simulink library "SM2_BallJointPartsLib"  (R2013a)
settings: Solver=ode45  StartTime=0.0  StopTime=10.0  RelTol=1e-3
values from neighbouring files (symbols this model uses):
  m = v*BEAM.rho    [FlexBeamModelConstruct2.m]    (also in FlexBeamModelConstruct3.m = BEAM.rho*v; FlexBeam_1D_Construct.m = REF.m/REF.l*a.*(linspace(1-OPT.MassBiais+1e-6,1+OPT.MassBiai; FlexBeam_3D_Construct.m = REF.m/REF.l*a.*(linspace(1-OPT.MassBiais+1e-6,1+OPT.MassBiai; FreeFlexBeam_3D_Construct.m = REF.m/REF.l*a.*tmp2)
  N = D(1)+(H4^2+H3^2)/H2^2-(E(1)*H4+F(1)*H3)/H2    [MGD.m]    (also in MGD2.m)
  s = -sign(imag(KGZ_fr_tmp))    [LinprogReguliOptimFunc_1.m]    (also in LinprogReguliOptimFunc_2.m; LinprogReguliOptimFunc_1 - Copie.m)
  X = cos(phi(i))*x+sin(phi(i))*y    [MGI.m]
  Y = fft(y(:,i),NFFT)/L    [fft_bis.m]    (also in MGI.m = -sin(phi(i))*x+cos(phi(i))*y)
  Z = z    [MGI.m]
undefined symbols (not defined in the file or in its folder): AxisID, deg, rad, SimParam
libraries: sm_lib x15

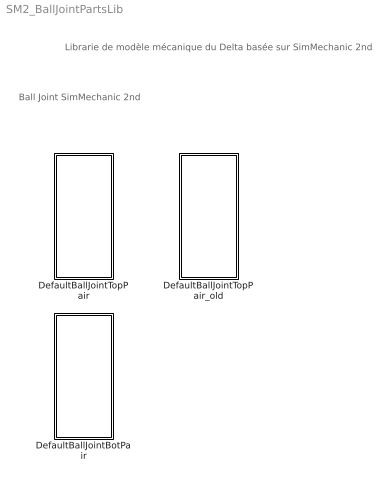
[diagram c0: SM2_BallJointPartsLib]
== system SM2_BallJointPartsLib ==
  note: Librarie de modèle mécanique du Delta basée sur SimMechanic 2nd
  note: Ball Joint SimMechanic 2nd
  DefaultBallJointBotPair : Subsystem  InitFcn=SimParam.BallJoint = Balljoint_paramInitFnc(RawParam);
  DefaultBallJointTopPair : Subsystem  InitFcn=SimParam.BallJoint = Balljoint_paramInitFnc(RawParam);
  DefaultBallJointTopPair_old : Subsystem  InitFcn=SimParam.BallJoint = Balljoint_paramInitFnc(RawParam);

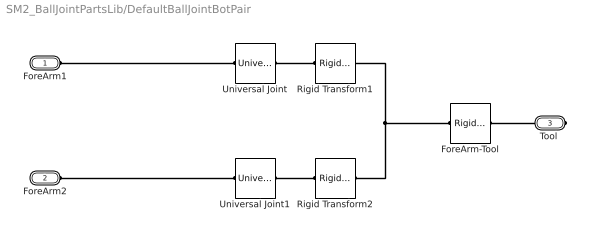
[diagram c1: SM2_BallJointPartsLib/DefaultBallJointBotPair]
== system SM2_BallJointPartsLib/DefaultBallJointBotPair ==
  ForeArm-Tool : sm_lib/Frames and  Transforms/Rigid  Transform  TranslationMethod=Cylindrical  TranslationLengthUnit=m  TranslationStandardAxis=+Z  TranslationStandardOffset=0  TranslationCartesianOffset=[-SimParam.BallJoint.r 0 0]  TranslationROffset=SimParam.BallJoint.r  TranslationROffsetUnits=m  TranslationZOffset=0  TranslationZOffsetUnits=m  TranslationThetaOffset=SimParam.BallJoint.Theta(AxisID)  TranslationThetaOffsetUnits=rad  RotationMethod=StandardAxis  RotationAngleUnits=rad  RotationStandardAxis=+Z  RotationAngle=SimParam.BallJoint.Theta(AxisID)  RotationArbitraryAxis=[1,1,1]  FollAlignAxisA=+X  BaseAlignAxisA=+Y  FollAlignAxisB=+Y  BaseAlignAxisB=+Z  BlockFunction=simmechanics.library.frames_transforms.rigid_transform
  Rigid Transform1 : sm_lib/Frames and  Transforms/Rigid  Transform  TranslationMethod=Cartesian  TranslationLengthUnit=m  TranslationStandardAxis=+Z  TranslationStandardOffset=0  TranslationCartesianOffset=[0 SimParam.BallJoint.d(2) 0]  TranslationROffset=0.2  TranslationROffsetUnits=m  TranslationZOffset=0  TranslationZOffsetUnits=m  TranslationThetaOffset=0  TranslationThetaOffsetUnits=deg  RotationMethod=None  RotationAngleUnits=rad  RotationStandardAxis=+Y  RotationAngle=0.2  RotationArbitraryAxis=[0 0 1]  FollAlignAxisA=+Z  BaseAlignAxisA=+Y  FollAlignAxisB=+X  BaseAlignAxisB=+X  BlockFunction=simmechanics.library.frames_transforms.rigid_transform
  Rigid Transform2 : sm_lib/Frames and  Transforms/Rigid  Transform  TranslationMethod=Cartesian  TranslationLengthUnit=m  TranslationStandardAxis=+Z  TranslationStandardOffset=0  TranslationCartesianOffset=[0 -SimParam.BallJoint.d(1) 0]  TranslationROffset=0.2  TranslationROffsetUnits=m  TranslationZOffset=0  TranslationZOffsetUnits=m  TranslationThetaOffset=0  TranslationThetaOffsetUnits=deg  RotationMethod=None  RotationAngleUnits=rad  RotationStandardAxis=+Y  RotationAngle=0.2  RotationArbitraryAxis=[0 0 1]  FollAlignAxisA=+Z  BaseAlignAxisA=+Y  FollAlignAxisB=+X  BaseAlignAxisB=+X  BlockFunction=simmechanics.library.frames_transforms.rigid_transform
  Universal Joint : sm_lib/Joints/Universal  Joint  SenseConstraintForceX=off  SenseConstraintForceY=off  SenseConstraintForceZ=off  SenseConstraintTorqueX=off  SenseConstraintTorqueY=off  SenseConstraintTorqueZ=off  ConstraintWrenchDir=FollowerOnBase  ConstraintWrenchFrame=BaseFrame  RxEquilibriumPosition=0  RxEquilibriumPositionUnits=deg  RxSpringStiffness=0  RxSpringStiffnessUnits=N*m/deg  RxDampingCoefficient=SimParam.BallJoint.c  RxDampingCoefficientUnits=N*m/(rad/s)  RxActuationMode=NoActuation  RxSensePosition=off  RxSenseVelocity=off  RxSenseAcceleration=off  RxSenseTorqueForce=off  RxPositionTargetValue=0  RxPositionTargetValueUnits=deg  RxPositionTargetSpecify=off  RxPositionTargetPriority=High  RxVelocityTargetValue=0  RxVelocityTargetValueUnits=deg/s  RxVelocityTargetSpecify=off  RxVelocityTargetPriority=High  RyEquilibriumPosition=0  RyEquilibriumPositionUnits=deg  RySpringStiffness=0  RySpringStiffnessUnits=N*m/deg  RyDampingCoefficient=SimParam.BallJoint.c  RyDampingCoefficientUnits=N*m/(rad/s)  RyActuationMode=NoActuation  RySensePosition=off  RySenseVelocity=off  RySenseAcceleration=off  RySenseTorqueForce=off  RyPositionTargetValue=0  RyPositionTargetValueUnits=deg  RyPositionTargetSpecify=off  RyPositionTargetPriority=High  RyVelocityTargetValue=0  RyVelocityTargetValueUnits=deg/s  RyVelocityTargetSpecify=off  RyVelocityTargetPriority=High  BlockFunction=simmechanics.library.joints.universal_joint
  Universal Joint1 : sm_lib/Joints/Universal  Joint  SenseConstraintForceX=off  SenseConstraintForceY=off  SenseConstraintForceZ=off  SenseConstraintTorqueX=off  SenseConstraintTorqueY=off  SenseConstraintTorqueZ=off  ConstraintWrenchDir=FollowerOnBase  ConstraintWrenchFrame=BaseFrame  RxEquilibriumPosition=0  RxEquilibriumPositionUnits=deg  RxSpringStiffness=0  RxSpringStiffnessUnits=N*m/deg  RxDampingCoefficient=SimParam.BallJoint.c  RxDampingCoefficientUnits=N*m/(rad/s)  RxActuationMode=NoActuation  RxSensePosition=off  RxSenseVelocity=off  RxSenseAcceleration=off  RxSenseTorqueForce=off  RxPositionTargetValue=0  RxPositionTargetValueUnits=deg  RxPositionTargetSpecify=off  RxPositionTargetPriority=High  RxVelocityTargetValue=0  RxVelocityTargetValueUnits=deg/s  RxVelocityTargetSpecify=off  RxVelocityTargetPriority=High  RyEquilibriumPosition=0  RyEquilibriumPositionUnits=deg  RySpringStiffness=0  RySpringStiffnessUnits=N*m/deg  RyDampingCoefficient=SimParam.BallJoint.c  RyDampingCoefficientUnits=N*m/(rad/s)  RyActuationMode=NoActuation  RySensePosition=off  RySenseVelocity=off  RySenseAcceleration=off  RySenseTorqueForce=off  RyPositionTargetValue=0  RyPositionTargetValueUnits=deg  RyPositionTargetSpecify=off  RyPositionTargetPriority=High  RyVelocityTargetValue=0  RyVelocityTargetValueUnits=deg/s  RyVelocityTargetSpecify=off  RyVelocityTargetPriority=High  BlockFunction=simmechanics.library.joints.universal_joint
  ForeArm1 : PMIOPort  Port=1  Side=Left
  ForeArm2 : PMIOPort  Port=2  Side=Left
  "Tool " : PMIOPort  Port=3  Side=Right
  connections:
  Universal Joint/LConn1 -- ForeArm1/RConn1
  Universal Joint1/LConn1 -- ForeArm2/RConn1
  ForeArm-Tool/LConn1 -- "Tool "/RConn1
  Rigid Transform2/LConn1 -- Rigid Transform1/LConn1 -- ForeArm-Tool/RConn1
  Rigid Transform2/RConn1 -- Universal Joint1/RConn1
  Rigid Transform1/RConn1 -- Universal Joint/RConn1

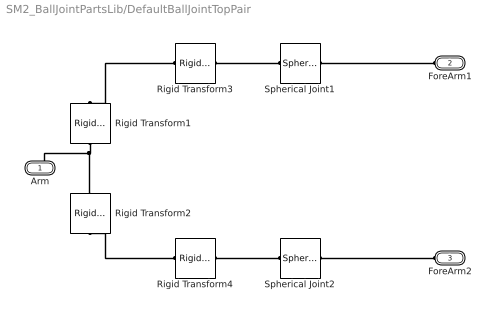
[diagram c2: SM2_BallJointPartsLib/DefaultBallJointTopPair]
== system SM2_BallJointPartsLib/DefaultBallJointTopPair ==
  Rigid Transform1 : sm_lib/Frames and  Transforms/Rigid  Transform  TranslationMethod=Cartesian  TranslationLengthUnit=m  TranslationStandardAxis=+Z  TranslationStandardOffset=0  TranslationCartesianOffset=[0 SimParam.BallJoint.d(1) 0]  TranslationROffset=0.2  TranslationROffsetUnits=m  TranslationZOffset=0  TranslationZOffsetUnits=m  TranslationThetaOffset=0  TranslationThetaOffsetUnits=deg  RotationMethod=None  RotationAngleUnits=rad  RotationStandardAxis=+Y  RotationAngle=0.2  RotationArbitraryAxis=[0 0 1]  FollAlignAxisA=+Z  BaseAlignAxisA=+Y  FollAlignAxisB=+X  BaseAlignAxisB=+X  BlockFunction=simmechanics.library.frames_transforms.rigid_transform
  Rigid Transform2 : sm_lib/Frames and  Transforms/Rigid  Transform  TranslationMethod=Cartesian  TranslationLengthUnit=m  TranslationStandardAxis=+Z  TranslationStandardOffset=0  TranslationCartesianOffset=[0 -SimParam.BallJoint.d(2) 0]  TranslationROffset=0.2  TranslationROffsetUnits=m  TranslationZOffset=0  TranslationZOffsetUnits=m  TranslationThetaOffset=0  TranslationThetaOffsetUnits=deg  RotationMethod=None  RotationAngleUnits=rad  RotationStandardAxis=+Y  RotationAngle=0.2  RotationArbitraryAxis=[0 0 1]  FollAlignAxisA=+Z  BaseAlignAxisA=+Y  FollAlignAxisB=+X  BaseAlignAxisB=+X  BlockFunction=simmechanics.library.frames_transforms.rigid_transform
  Rigid Transform3 : sm_lib/Frames and  Transforms/Rigid  Transform  TranslationMethod=None  TranslationLengthUnit=m  TranslationStandardAxis=+Z  TranslationStandardOffset=0  TranslationCartesianOffset=[0 -SimParam.BallJoint.d(2) 0]  TranslationROffset=0.2  TranslationROffsetUnits=m  TranslationZOffset=0  TranslationZOffsetUnits=m  TranslationThetaOffset=0  TranslationThetaOffsetUnits=deg  RotationMethod=ArbitraryAxis  RotationAngleUnits=rad  RotationStandardAxis=+Y  RotationAngle=SimParam.IC.ArmForeArmRotAng(AxisID)  RotationArbitraryAxis=SimParam.IC.ArmForeArmRotVec(AxisID,:)  FollAlignAxisA=+Z  BaseAlignAxisA=+Y  FollAlignAxisB=+X  BaseAlignAxisB=+X  BlockFunction=simmechanics.library.frames_transforms.rigid_transform
  Rigid Transform4 : sm_lib/Frames and  Transforms/Rigid  Transform  TranslationMethod=None  TranslationLengthUnit=m  TranslationStandardAxis=+Z  TranslationStandardOffset=0  TranslationCartesianOffset=[0 -SimParam.BallJoint.d(2) 0]  TranslationROffset=0.2  TranslationROffsetUnits=m  TranslationZOffset=0  TranslationZOffsetUnits=m  TranslationThetaOffset=0  TranslationThetaOffsetUnits=deg  RotationMethod=ArbitraryAxis  RotationAngleUnits=rad  RotationStandardAxis=+Y  RotationAngle=SimParam.IC.ArmForeArmRotAng(AxisID)  RotationArbitraryAxis=SimParam.IC.ArmForeArmRotVec(AxisID,:)  FollAlignAxisA=+Z  BaseAlignAxisA=+Y  FollAlignAxisB=+X  BaseAlignAxisB=+X  BlockFunction=simmechanics.library.frames_transforms.rigid_transform
  Spherical Joint1 : sm_lib/Joints/Spherical  Joint  SenseConstraintForceX=off  SenseConstraintForceY=off  SenseConstraintForceZ=off  SenseConstraintTorqueX=off  SenseConstraintTorqueY=off  SenseConstraintTorqueZ=off  ConstraintWrenchDir=FollowerOnBase  ConstraintWrenchFrame=BaseFrame  DefPosRotationMethod=None  DefPosRotationAngleUnits=deg  DefPosRotationStandardAxis=+Z  DefPosRotationAngle=0  DefPosRotationArbitraryAxis=[0 0 1]  DefPosFollAlignAxisA=+X  DefPosBaseAlignAxisA=+Y  DefPosFollAlignAxisB=+Y  DefPosBaseAlignAxisB=+Z  EqPosRotationMethod=None  EqPosRotationAngleUnits=deg  EqPosRotationStandardAxis=+Z  EqPosRotationAngle=0  EqPosRotationArbitraryAxis=[0 0 1]  EqPosFollAlignAxisA=+X  EqPosBaseAlignAxisA=+Y  EqPosFollAlignAxisB=+Y  EqPosBaseAlignAxisB=+Z  SpringStiffness=0  SpringStiffnessUnits=N*m/deg  DampingCoefficient=SimParam.BallJoint.c  DampingCoefficientUnits=N*m/(rad/s)  ActuateTorqueX=off  ActuateTorqueY=off  ActuateTorqueZ=off  ActuateTorque=off  ActuationMode=NoActuation  ActuationFrame=BaseFrame  SensePosition=off  SenseVelocityX=off  SenseVelocityY=off  SenseVelocityZ=off  SenseVelocity=off  SenseAccelerationX=off  SenseAccelerationY=off  SenseAccelerationZ=off  SenseAcceleration=off  SenseTorqueX=off  SenseTorqueY=off  SenseTorqueZ=off  SenseTorqueForce=off  SensingFrame=BaseFrame  PositionTargetRotationMethod=StandardAxis  PositionTargetRotationAngleUnits=rad  PositionTargetRotationStandardAxis=+Z  PositionTargetRotationAngle=0  PositionTargetRotationArbitraryAxis=SimParam.IC.ArmForeArmRotVec(AxisID,:)  PositionTargetFollAlignAxisA=+X  PositionTargetBaseAlignAxisA=+Y  PositionTargetFollAlignAxisB=+Y  PositionTargetBaseAlignAxisB=+Z  PositionTargetSpecify=off  PositionTargetPriority=Low  VelocityTargetValue=[0 0 0]  VelocityTargetValueUnits=rad/s  VelocityTargetSpecify=on  VelocityTargetPriority=High  VelocityTargetInFollowerFrame=on  BlockFunction=simmechanics.library.joints.spherical_joint
  Spherical Joint2 : sm_lib/Joints/Spherical  Joint  SenseConstraintForceX=off  SenseConstraintForceY=off  SenseConstraintForceZ=off  SenseConstraintTorqueX=off  SenseConstraintTorqueY=off  SenseConstraintTorqueZ=off  ConstraintWrenchDir=FollowerOnBase  ConstraintWrenchFrame=BaseFrame  DefPosRotationMethod=None  DefPosRotationAngleUnits=deg  DefPosRotationStandardAxis=+Z  DefPosRotationAngle=0  DefPosRotationArbitraryAxis=[0 0 1]  DefPosFollAlignAxisA=+X  DefPosBaseAlignAxisA=+Y  DefPosFollAlignAxisB=+Y  DefPosBaseAlignAxisB=+Z  EqPosRotationMethod=None  EqPosRotationAngleUnits=deg  EqPosRotationStandardAxis=+Z  EqPosRotationAngle=0  EqPosRotationArbitraryAxis=[0 0 1]  EqPosFollAlignAxisA=+X  EqPosBaseAlignAxisA=+Y  EqPosFollAlignAxisB=+Y  EqPosBaseAlignAxisB=+Z  SpringStiffness=0  SpringStiffnessUnits=N*m/deg  DampingCoefficient=SimParam.BallJoint.c  DampingCoefficientUnits=N*m/(rad/s)  ActuateTorqueX=off  ActuateTorqueY=off  ActuateTorqueZ=off  ActuateTorque=off  ActuationMode=NoActuation  ActuationFrame=BaseFrame  SensePosition=off  SenseVelocityX=off  SenseVelocityY=off  SenseVelocityZ=off  SenseVelocity=off  SenseAccelerationX=off  SenseAccelerationY=off  SenseAccelerationZ=off  SenseAcceleration=off  SenseTorqueX=off  SenseTorqueY=off  SenseTorqueZ=off  SenseTorqueForce=off  SensingFrame=BaseFrame  PositionTargetRotationMethod=StandardAxis  PositionTargetRotationAngleUnits=rad  PositionTargetRotationStandardAxis=+Z  PositionTargetRotationAngle=0  PositionTargetRotationArbitraryAxis=SimParam.IC.ArmForeArmRotVec(AxisID,:)  PositionTargetFollAlignAxisA=+X  PositionTargetBaseAlignAxisA=+Y  PositionTargetFollAlignAxisB=+Y  PositionTargetBaseAlignAxisB=+Z  PositionTargetSpecify=off  PositionTargetPriority=Low  VelocityTargetValue=[0 0 0]  VelocityTargetValueUnits=rad/s  VelocityTargetSpecify=on  VelocityTargetPriority=High  VelocityTargetInFollowerFrame=on  BlockFunction=simmechanics.library.joints.spherical_joint
  Arm : PMIOPort  Port=1  Side=Right
  ForeArm1 : PMIOPort  Port=2  Side=Left
  ForeArm2 : PMIOPort  Port=3  Side=Left
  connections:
  Rigid Transform1/LConn1 -- Arm/RConn1 -- Rigid Transform2/LConn1
  Spherical Joint1/LConn1 -- Rigid Transform3/RConn1
  ForeArm2/RConn1 -- Spherical Joint2/RConn1
  Rigid Transform4/RConn1 -- Spherical Joint2/LConn1
  Rigid Transform3/LConn1 -- Rigid Transform1/RConn1
  Rigid Transform4/LConn1 -- Rigid Transform2/RConn1
  ForeArm1/RConn1 -- Spherical Joint1/RConn1

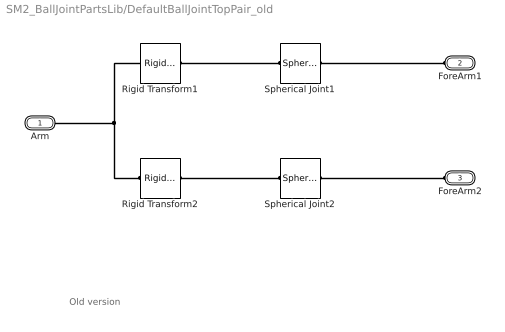
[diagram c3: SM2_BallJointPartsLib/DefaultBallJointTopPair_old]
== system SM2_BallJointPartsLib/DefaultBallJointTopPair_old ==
  note: Old version
  Rigid Transform1 : sm_lib/Frames and  Transforms/Rigid  Transform  TranslationMethod=Cartesian  TranslationLengthUnit=m  TranslationStandardAxis=+Z  TranslationStandardOffset=0  TranslationCartesianOffset=[0 SimParam.BallJoint.d(1) 0]  TranslationROffset=0.2  TranslationROffsetUnits=m  TranslationZOffset=0  TranslationZOffsetUnits=m  TranslationThetaOffset=0  TranslationThetaOffsetUnits=deg  RotationMethod=None  RotationAngleUnits=rad  RotationStandardAxis=+Y  RotationAngle=0.2  RotationArbitraryAxis=[0 0 1]  FollAlignAxisA=+Z  BaseAlignAxisA=+Y  FollAlignAxisB=+X  BaseAlignAxisB=+X  BlockFunction=simmechanics.library.frames_transforms.rigid_transform
  Rigid Transform2 : sm_lib/Frames and  Transforms/Rigid  Transform  TranslationMethod=Cartesian  TranslationLengthUnit=m  TranslationStandardAxis=+Z  TranslationStandardOffset=0  TranslationCartesianOffset=[0 -SimParam.BallJoint.d(2) 0]  TranslationROffset=0.2  TranslationROffsetUnits=m  TranslationZOffset=0  TranslationZOffsetUnits=m  TranslationThetaOffset=0  TranslationThetaOffsetUnits=deg  RotationMethod=None  RotationAngleUnits=rad  RotationStandardAxis=+Y  RotationAngle=0.2  RotationArbitraryAxis=[0 0 1]  FollAlignAxisA=+Z  BaseAlignAxisA=+Y  FollAlignAxisB=+X  BaseAlignAxisB=+X  BlockFunction=simmechanics.library.frames_transforms.rigid_transform
  Spherical Joint1 : sm_lib/Joints/Spherical  Joint  SenseConstraintForceX=off  SenseConstraintForceY=off  SenseConstraintForceZ=off  SenseConstraintTorqueX=off  SenseConstraintTorqueY=off  SenseConstraintTorqueZ=off  ConstraintWrenchDir=FollowerOnBase  ConstraintWrenchFrame=BaseFrame  DefPosRotationMethod=None  DefPosRotationAngleUnits=deg  DefPosRotationStandardAxis=+Z  DefPosRotationAngle=0  DefPosRotationArbitraryAxis=[0 0 1]  DefPosFollAlignAxisA=+X  DefPosBaseAlignAxisA=+Y  DefPosFollAlignAxisB=+Y  DefPosBaseAlignAxisB=+Z  EqPosRotationMethod=None  EqPosRotationAngleUnits=deg  EqPosRotationStandardAxis=+Z  EqPosRotationAngle=0  EqPosRotationArbitraryAxis=[0 0 1]  EqPosFollAlignAxisA=+X  EqPosBaseAlignAxisA=+Y  EqPosFollAlignAxisB=+Y  EqPosBaseAlignAxisB=+Z  SpringStiffness=0  SpringStiffnessUnits=N*m/deg  DampingCoefficient=SimParam.BallJoint.c  DampingCoefficientUnits=N*m/(rad/s)  ActuateTorqueX=off  ActuateTorqueY=off  ActuateTorqueZ=off  ActuateTorque=off  ActuationMode=NoActuation  ActuationFrame=BaseFrame  SensePosition=off  SenseVelocityX=off  SenseVelocityY=off  SenseVelocityZ=off  SenseVelocity=off  SenseAccelerationX=off  SenseAccelerationY=off  SenseAccelerationZ=off  SenseAcceleration=off  SenseTorqueX=off  SenseTorqueY=off  SenseTorqueZ=off  SenseTorqueForce=off  SensingFrame=BaseFrame  PositionTargetRotationMethod=ArbitraryAxis  PositionTargetRotationAngleUnits=rad  PositionTargetRotationStandardAxis=+Z  PositionTargetRotationAngle=SimParam.IC.ArmForeArmRotAng(AxisID)  PositionTargetRotationArbitraryAxis=SimParam.IC.ArmForeArmRotVec(AxisID,:)  PositionTargetFollAlignAxisA=+X  PositionTargetBaseAlignAxisA=+Y  PositionTargetFollAlignAxisB=+Y  PositionTargetBaseAlignAxisB=+Z  PositionTargetSpecify=on  PositionTargetPriority=High  VelocityTargetValue=[0 0 0]  VelocityTargetValueUnits=rad/s  VelocityTargetSpecify=on  VelocityTargetPriority=High  VelocityTargetInFollowerFrame=on  BlockFunction=simmechanics.library.joints.spherical_joint
  Spherical Joint2 : sm_lib/Joints/Spherical  Joint  SenseConstraintForceX=off  SenseConstraintForceY=off  SenseConstraintForceZ=off  SenseConstraintTorqueX=off  SenseConstraintTorqueY=off  SenseConstraintTorqueZ=off  ConstraintWrenchDir=FollowerOnBase  ConstraintWrenchFrame=BaseFrame  DefPosRotationMethod=None  DefPosRotationAngleUnits=deg  DefPosRotationStandardAxis=+Z  DefPosRotationAngle=0  DefPosRotationArbitraryAxis=[0 0 1]  DefPosFollAlignAxisA=+X  DefPosBaseAlignAxisA=+Y  DefPosFollAlignAxisB=+Y  DefPosBaseAlignAxisB=+Z  EqPosRotationMethod=None  EqPosRotationAngleUnits=deg  EqPosRotationStandardAxis=+Z  EqPosRotationAngle=0  EqPosRotationArbitraryAxis=[0 0 1]  EqPosFollAlignAxisA=+X  EqPosBaseAlignAxisA=+Y  EqPosFollAlignAxisB=+Y  EqPosBaseAlignAxisB=+Z  SpringStiffness=0  SpringStiffnessUnits=N*m/deg  DampingCoefficient=SimParam.BallJoint.c  DampingCoefficientUnits=N*m/(rad/s)  ActuateTorqueX=off  ActuateTorqueY=off  ActuateTorqueZ=off  ActuateTorque=off  ActuationMode=NoActuation  ActuationFrame=BaseFrame  SensePosition=off  SenseVelocityX=off  SenseVelocityY=off  SenseVelocityZ=off  SenseVelocity=off  SenseAccelerationX=off  SenseAccelerationY=off  SenseAccelerationZ=off  SenseAcceleration=off  SenseTorqueX=off  SenseTorqueY=off  SenseTorqueZ=off  SenseTorqueForce=off  SensingFrame=BaseFrame  PositionTargetRotationMethod=ArbitraryAxis  PositionTargetRotationAngleUnits=rad  PositionTargetRotationStandardAxis=+Z  PositionTargetRotationAngle=SimParam.IC.ArmForeArmRotAng(AxisID)  PositionTargetRotationArbitraryAxis=SimParam.IC.ArmForeArmRotVec(AxisID,:)  PositionTargetFollAlignAxisA=+X  PositionTargetBaseAlignAxisA=+Y  PositionTargetFollAlignAxisB=+Y  PositionTargetBaseAlignAxisB=+Z  PositionTargetSpecify=on  PositionTargetPriority=High  VelocityTargetValue=[0 0 0]  VelocityTargetValueUnits=rad/s  VelocityTargetSpecify=on  VelocityTargetPriority=High  VelocityTargetInFollowerFrame=on  BlockFunction=simmechanics.library.joints.spherical_joint
  Arm : PMIOPort  Port=1  Side=Right
  ForeArm1 : PMIOPort  Port=2  Side=Left
  ForeArm2 : PMIOPort  Port=3  Side=Left
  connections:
  Rigid Transform2/LConn1 -- Rigid Transform1/LConn1 -- Arm/RConn1
  Spherical Joint1/LConn1 -- Rigid Transform1/RConn1
  Spherical Joint2/LConn1 -- Rigid Transform2/RConn1
  ForeArm1/RConn1 -- Spherical Joint1/RConn1
  Spherical Joint2/RConn1 -- ForeArm2/RConn1
